FUNCTION_BLOCK FB 1
BEGIN
	L		W#16#4321
	T		MW 0
END_FUNCTION_BLOCK


FUNCTION FC 1 : VOID
BEGIN
	L		W#16#1234
	T		MW 0
	CALL		FC 2
END_FUNCTION


FUNCTION FC 2 : VOID
BEGIN
	L		W#16#6789
	T		MW 0
	L		10
	T		LB 0
END_FUNCTION


FUNCTION FC 3 : VOID
BEGIN
	L		1
	T		LB 0
	CALL		FC 2
	__ASSERT==	LB 0,	1
END_FUNCTION


FUNCTION FC 4 : VOID
VAR_INPUT
	INPVAR		: INT
END_VAR
BEGIN
	L		#INPVAR
	__ASSERT==	__ACCU 1,	9976
END_FUNCTION


FUNCTION FC 5 : VOID
VAR_INPUT
	INPVAR2		: INT
END_VAR
BEGIN
	CALL FC 4 (
		INPVAR		:= #INPVAR2,	// This is a parameter
	)
END_FUNCTION


FUNCTION FC 6 : VOID
BEGIN
	// Only check OV and OS bits
	__ASSERT==	__STW OV,	1
	__ASSERT==	__STW OS,	0
	L		1
	L		1
	+I
	__ASSERT==	__STW OV,	0
	__ASSERT==	__STW OS,	0
END_FUNCTION


FUNCTION FC 7 : VOID
BEGIN
	// Trigger an overflow
	__ASSERT==	__STW OV,	0
	__ASSERT==	__STW OS,	0
	L		30000
	L		30000
	+I
	__ASSERT==	__STW OV,	1
	__ASSERT==	__STW OS,	1
END_FUNCTION


ORGANIZATION_BLOCK OB 1
BEGIN
	CALL		FC 1
	__ASSERT==	MW 0,	W#16#6789
	L		0
	T		MW 0
	__ASSERT==	MW 0,	0
	UC		FC 1
	__ASSERT==	MW 0,	W#16#6789
	L		0
	T		MW 0
	__ASSERT==	MW 0,	0
	SET
	CC		FC 1
	__ASSERT==	MW 0,	W#16#6789
	L		0
	T		MW 0
	__ASSERT==	MW 0,	0
	CLR
	CC		FC 1
	__ASSERT==	MW 0,	0

	// Test localdata stack
	L		255
	T		LB 0
	__ASSERT==	LB 0,	255
	CALL		FC 3
	__ASSERT==	LB 0,	255

	CALL FC 5 (
		INPVAR2		:= 9976,
	)

	// Test OV/OS bits over call boundaries
	__STWRST
	L		30000
	L		30000
	+I
	__ASSERT==	__STW OV,	1
	__ASSERT==	__STW OS,	1
	CALL FC 6
	__ASSERT==	__STW OV,	0
	__ASSERT==	__STW OS,	0
	__STWRST
	CALL FC 7
	__ASSERT==	__STW OV,	1
	__ASSERT==	__STW OS,	0


	// Test raw FB call
	UC		FB 1
	SET
	CC		FB 1


	// Test indirect calls
	L		0
	T		MW 0
	L		1
	T		MW 50
	CLR
	UC		FC [MW 50]
	L		MW 0
	__ASSERT==	__ACCU 1,	W#16#6789
	L		0
	T		MW 0
	SET
	CC		FC [MW 50]
	L		MW 0
	__ASSERT==	__ACCU 1,	W#16#6789
	L		0
	T		MW 0
	CLR
	UC		FB [MW 50]
	L		MW 0
	__ASSERT==	__ACCU 1,	W#16#4321
	L		0
	T		MW 0
	SET
	CC		FB [MW 50]
	L		MW 0
	__ASSERT==	__ACCU 1,	W#16#4321

END_ORGANIZATION_BLOCK
